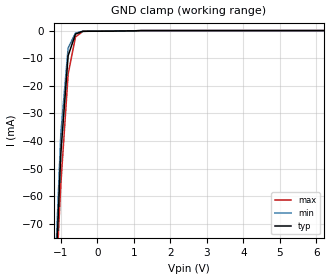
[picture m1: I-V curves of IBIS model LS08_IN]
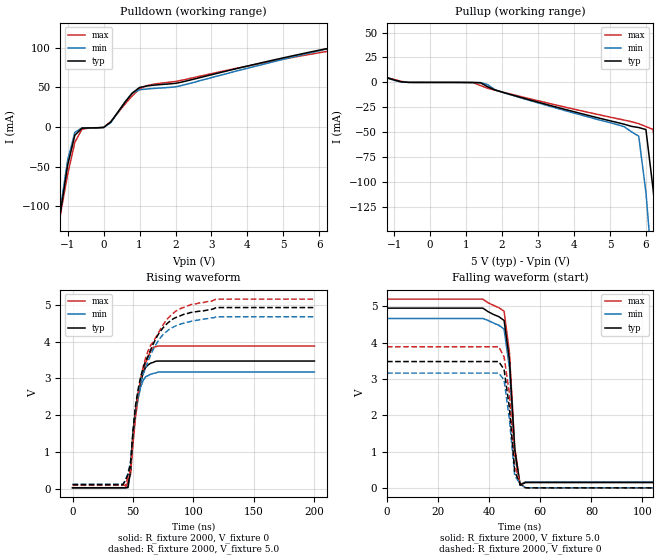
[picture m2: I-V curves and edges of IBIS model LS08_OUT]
|   TEXAS INSTRUMENTS INCORPORATED
|   Standard Linear and Logic
|   IBIS Model of SN74LS08
|   QUADRUPLE 2-INPUT POSITIVE-AND GATES
|   SOIC 14-pin (D),SSOP 14-pin (DB), 14-pin PDIP (N), SOP 14-pin (NS)
[IBIS Ver]   3.2
[Comment Char]  |_char
[File Name]   sn74ls08.ibs
[File Rev]   3.2 | i_die
[Date]   Nov.12, 2004
[Source]   File originated at Texas Instruments, Inc.
[Notes]   The following is a sample IBIS file for the SN74LS08.
   - FILE REV HISTORY
   - 3.2 Re-Release IBIS file on 11/16/04
   - Power clamp data deleted as there is no power-clamp diode.
   - All test data contained in this file are derived from
   actual measurement.
   - The measurement used NS package.
   - We have data across voltage and temperature, but not across
   process.
   - File created by Nobuhisa Ohtsubo, TIJ SLL Product Engineering.
[Disclaimer] Property of Texas Instruments Incorporated. Unauthorized
   reproduction and/or distribution is strictly prohibited.
   This product is protected under copyright law.
   Created 2000, (C) Copyright 2000, Texas Instruments Inc.,
   All Rights Reserved.
   UNLESS THERE IS A SIGNED, WRITTEN AGREEMENT TO THE
   CONTRARY, TEXAS INSTRUMENTS (TI) IS PROVIDING THE IBIS
   MODELS AND WITHOUT ANY WARRANTY, EXPRESSED OR
   IMPLIED. TI assumes no liability for:
   1) the accuracy of the IBIS models provided to your
   company;
   2) the proper functioning of these IBIS Models in your
   design or for any resulting applications; or
   3) infringement of patents, copyrights or intellectual
   property rights resulting from your use of these IBIS
   models.
   TI provides IBIS Models as a service to our customers.
   You and your company shall not distribute, sell or give
   these models to anyone else without prior written
   permission from TI.
   TI reserves the right to make changes to our products or
   to discontinue any semiconductor product or service
   without notice, and advises our customers to obtain the
   latest version of relevant information to verify, before
   placing orders, that the information being relied on is
   current.
   Please be aware that your receipt and use of the IBIS
   information provided shall serve as acceptance of these
   terms and conditions. If you do not accept these terms,
   you should return or destroy the IBIS models and any
   other accompanying information immediately.
| Component LS08_D 14-pin SOIC
[Component]   LS08_D
[Manufacturer]  Texas Instruments, Inc.
[Package]
|   typ   min   max
R_pkg   0.031   0.028   0.034
L_pkg   3.109nH   2.462nH   3.889nH
C_pkg   0.473pF   0.363pF   0.628pF
[Pin]   signal_name   model_name   R_pin   L_pin   C_pin
1   1A   LS08_IN   0.033   3.854nH   0.622pF
2   1B   LS08_IN   0.032   3.188nH   0.473pF
3   1Y   LS08_OUT   0.028   2.462nH   0.377pF
4   2A   LS08_IN   0.031   2.596nH   0.363pF
5   2B   LS08_IN   0.028   2.521nH   0.372pF
6   2Y   LS08_OUT   0.034   3.250nH   0.476pF
7   GND   GND   0.034   3.889nH   0.628pF
8   3Y   LS08_OUT   0.034   3.889nH   0.628pF
9   3A   LS08_IN   0.034   3.250nH   0.476pF
10   3B   LS08_IN   0.028   2.521nH   0.372pF
11   4Y   LS08_OUT   0.031   2.596nH   0.364pF
12   4A   LS08_IN   0.028   2.462nH   0.377pF
13   4B   LS08_IN   0.032   3.188nH   0.473pF
14   VCC   POWER   0.033   3.854nH   0.622pF
| Component LS08_DB 14-pin SSOP
[Component]   LS08_DB
[Manufacturer]  Texas Instruments, Inc.
[Package]
|   typ   min   max
R_pkg   0.044   0.041   0.046
L_pkg   3.551nH   3.258nH   3.927nH
C_pkg   0.402pF   0.360pF   0.421pF
[Pin]   signal_name   model_name   R_pin   L_pin   C_pin
1   1A   LS08_IN   0.046   3.927nH   0.408pF
2   1B   LS08_IN   0.044   3.587nH   0.421pF
3   1Y   LS08_OUT   0.041   3.289nH   0.398pF
4   2A   LS08_IN   0.042   3.258nH   0.360pF
5   2B   LS08_IN   0.041   3.286nH   0.403pF
6   2Y   LS08_OUT   0.044   3.586nH   0.421pF
7   GND   GND   0.046   3.927nH   0.408pF
8   3Y   LS08_OUT   0.046   3.927nH   0.408pF
9   3A   LS08_IN   0.044   3.586nH   0.421pF
10   3B   LS08_IN   0.041   3.286nH   0.403pF
11   4Y   LS08_OUT   0.043   3.258nH   0.360pF
12   4A   LS08_IN   0.041   3.289nH   0.398pF
13   4B   LS08_IN   0.044   3.587nH   0.421pF
14   VCC   POWER   0.046   3.927nH   0.408pF
| Component LS08_N 14-pin PDIP
[Component]   LS08_N
[Manufacturer]   Texas Instruments, Inc.
[Package]
|   typ   min   max
R_pkg   4.500e-02   3.700e-02   6.300e-02
L_pkg   5.407e-09   3.922e-09   6.942e-09
C_pkg   3.890e-13   2.050e-13   6.040e-13
[Pin]   signal_name   model_name   R_pin   L_pin   C_pin
1   1A   LS08_IN   6.300e-02   6.942e-09   6.040e-13
2   1B   LS08_IN   3.700e-02   6.200e-09   4.060e-13
3   1Y   LS08_OUT   4.200e-02   4.389e-09   3.220e-13
4   2A   LS08_IN   3.800e-02   3.922e-09   2.050e-13
5   2B   LS08_IN   3.900e-02   4.301e-09   2.980e-13
6   2Y   LS08_OUT   3.800e-02   5.329e-09   3.560e-13
7   GND   GND   5.300e-02   6.510e-09   5.440e-13
8   3Y   LS08_OUT   5.300e-02   6.437e-09   5.390e-13
9   3A   LS08_IN   3.900e-02   5.352e-09   3.470e-13
10   3B   LS08_IN   4.200e-02   4.473e-09   2.970e-13
11   4Y   LS08_OUT   4.400e-02   4.326e-09   2.250e-13
12   4A   LS08_IN   4.200e-02   4.295e-09   2.800e-13
13   4B   LS08_IN   4.200e-02   6.318e-09   4.180e-13
14   VCC   POWER   6.100e-02   6.900e-09   6.030e-13
| Component LS08_NS 14-pin SOP
[Component]   LS08_NS
[Manufacturer]  Texas Instruments, Inc.
[Package]
|   typ   min   max
R_pkg   0.045   0.039   0.054
L_pkg   3.796nH   2.561nH   4.952nH
C_pkg   0.528pF   0.288pF   0.710pF
[Pin]   signal_name   model_name   R_pin   L_pin   C_pin
1   1A   LS08_IN   0.047   4.867nH   0.706pF
2   1B   LS08_IN   0.051   4.083nH   0.592pF
3   1Y   LS08_OUT   0.041   2.915nH   0.376pF
4   2A   LS08_IN   0.039   2.561nH   0.288pF
5   2B   LS08_IN   0.041   3.101nH   0.430pF
6   2Y   LS08_OUT   0.047   4.047nH   0.589pF
7   GND   GND   0.051   4.909nH   0.700pF
8   3Y   LS08_OUT   0.045   4.784nH   0.694pF
9   3A   LS08_IN   0.054   4.176nH   0.597pF
10   3B   LS08_IN   0.039   3.287nH   0.449pF
11   4Y   LS08_OUT   0.039   2.586nH   0.294pF
12   4A   LS08_IN   0.040   2.802nH   0.371pF
13   4B   LS08_IN   0.049   4.080nH   0.593pF
14   VCC   POWER   0.052   4.952nH   0.710pF
| Models and submodels in the file (2): LS08_IN (Input), LS08_OUT (Output)
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| Model LS08_IN
[Model]   LS08_IN
Model_type  Input
Polarity   Inverting
Vinl = 0.8
Vinh = 2.0
| variable   typ   min   max
C_comp   1.33pf   1.00pf   1.66pf
[Temperature Range]   25   0   70
[Voltage Range]   5.0   4.75   5.25
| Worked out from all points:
|   GND clamp passes 1 mA (typ) near -0.54 V on its own axis
[GND Clamp]
|   Voltage   I(typ)   I(min)   I(max)
-5V       -1.743A    -1.862A    -1.563A
-1.2V     -107.8mA   -101.5mA   -110mA
-1V       -44.46mA   -37.32mA   -55.68mA
-800mV    -9.117mA   -6.302mA   -15.81mA
-600mV    -1.293mA   -947.5uA   -2.367mA
-400mV    -253.3uA   -256.3uA   -300.8uA
-200mV    -236.5uA   -244.5uA   -213.9uA
10V       12.74nA    11.36nA    18.89nA
|  Model LS08_OUT
[Model]   LS08_OUT
Model_type  Output
Polarity   Non-Inverting
Vmeas = 1.3v
Cref = 15pf
Rref = 2000
Vref = 0V
| variable   typ   min   max
C_comp   5.8pf   4.35pf   7.25pf
[Temperature Range]   25   0   70
[Voltage Range]   5.0   4.75   5.25
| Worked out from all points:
|   slope of the pulldown table from 0 to 0.75 V, typ, clamps not added: 18.4 ohm
|   slope of the pullup table from 0 to 0.75 V, typ, clamps not added: 34 kohm
|   rising waveform, R_fixture 2000, V_fixture 0: 20-80 % time 7.12ns typ, 6.53ns min, 8.96ns max; typ from 0.022 V to 3.47 V
|   falling waveform, R_fixture 2000, V_fixture 5.0: 20-80 % time 2.91ns typ, 2.91ns min, 2.89ns max; typ from 4.95 V to 0.156 V
|   rising waveform, R_fixture 2000, V_fixture 5.0: 20-80 % time 18.3ns typ, 17.6ns min, 19.9ns max; typ from 0.11 V to 4.93 V
|   falling waveform, R_fixture 2000, V_fixture 0: 20-80 % time 2.93ns typ, 2.92ns min, 3.01ns max; typ from 3.48 V to 0.011 V
[Pulldown]
|   Voltage   I(typ)   I(min)   I(max)
-5V       -1.674A    -1.769A    -1.5A
-1.4V     -194.6mA   -189.3mA   -196.9mA
-1.2V     -108mA     -102.4mA   -110mA
-1V       -48.29mA   -41.91mA   -59.95mA
-800mV    -10.55mA   -6.927mA   -19.36mA
-600mV    -1.523mA   -1.226mA   -2.886mA
99.48fV   -671.3uA   -751uA     -520.3uA
1V        49.81mA    46.87mA    47.86mA
2V        55mA       50.56mA    57.35mA
6.6V      102.4mA    102.2mA    98.22mA
8V        115.2mA    126.8mA    108.8mA
10V       133.6mA    164.4mA    124mA
[Pullup]
|   Voltage   I(typ)   I(min)   I(max)
-5V       51.08mA    53.71mA    46.39mA
-1V       2.456mA    2.167mA    2.908mA
1.2V      -103.5uA   -102.1uA   -265.5uA
1.4V      -393.9uA   -152.7uA   -3.186mA
2V        -9.733mA   -9.726mA   -9.591mA
5.4V      -41.96mA   -44.5mA    -37.8mA
5.8V      -45.25mA   -53.86mA   -41.39mA
6V        -47.28mA   -110mA     -44.26mA
6.2V      -107.1mA   -197.5mA   -47.16mA
6.4V      -180.1mA   -296.9mA   -100.6mA
6.6V      -274.5mA   -387.2mA   -165.8mA
10V       -1.695A    -1.904A    -1.423A
[Ramp]
| variable   typ   min   max
dV/dt_r  2.124E-00/7.397E-09  1.914E-00/6.550E-09  2.370E-00/9.531E-09
dV/dt_f  2.982E+00/2.178E-09  2.818E+00/2.224E-09  3.144E+00/2.311E-09
R_load = 2000
[Rising Waveform]
R_fixture = 2000
V_fixture = 0
V_fixture_min = 0
V_fixture_max = 0
C_fixture = 0pf
L_fixture = 0nH
|   Time   V(typ)   V(min)   V(max)
0s        21.98mV    23.41mV    20.04mV
43.75ns   22.44mV    24.19mV    20.18mV
45.83ns   32.5mV     26.19mV    189.7mV
47.92ns   507.3mV    483.6mV    378.3mV
50ns      1.494V     1.469V     1.233V
52.08ns   2.151V     2.099V     1.945V
56.25ns   2.906V     2.754V     2.858V
60.42ns   3.302V     3.047V     3.419V
66.67ns   3.437V     3.136V     3.844V
200ns     3.474V     3.176V     3.883V
[Falling Waveform]
R_fixture = 2000
V_fixture = 5.0
V_fixture_min = 4.75
V_fixture_max = 5.25
C_fixture = 0pf
L_fixture = 0nH
|   Time   V(typ)   V(min)   V(max)
0s        4.951V     4.666V     5.198V
37.5ns    4.951V     4.666V     5.198V
39.58ns   4.853V     4.612V     5.096V
43.75ns   4.717V     4.481V     4.963V
45.83ns   4.612V     4.377V     4.868V
47.92ns   3.541V     3.309V     3.73V
50ns      1.058V     992.8mV    1.131V
52.08ns   83.54mV    86.14mV    108.1mV
54.17ns   156mV      172.4mV    166.7mV
200ns     156mV      172.4mV    166.7mV
[Rising Waveform]
R_fixture = 2000
V_fixture = 5.0
V_fixture_min = 4.75
V_fixture_max = 5.25
C_fixture = 0pf
L_fixture = 0nH
|   Time   V(typ)   V(min)   V(max)
0s        110.1mV    116.9mV    89mV
43.75ns   223.4mV    228.2mV    89.85mV
47.92ns   676.2mV    731.1mV    483.5mV
52.08ns   2.26V      2.217V     2.067V
56.25ns   3.031V     2.886V     2.983V
60.42ns   3.471V     3.287V     3.557V
72.92ns   4.296V     4.122V     4.358V
85.42ns   4.659V     4.433V     4.834V
118.8ns   4.931V     4.679V     5.16V
200ns     4.931V     4.679V     5.16V
[Falling Waveform]
R_fixture = 2000
V_fixture = 0
V_fixture_min = 0
V_fixture_max = 0
C_fixture = 0pf
L_fixture = 0nH
|   Time   V(typ)   V(min)   V(max)
0s        3.482V     3.165V     3.889V
43.75ns   3.482V     3.165V     3.889V
45.83ns   3.265V     2.978V     3.609V
47.92ns   2.207V     1.891V     2.605V
50ns      451.3mV    348.9mV    663.8mV
52.08ns   125.5mV    120.8mV    139.2mV
54.17ns   12.31mV    12.58mV    14.21mV
56.25ns   11.04mV    12.44mV    13.22mV
200ns     11.04mV    12.44mV    13.22mV
